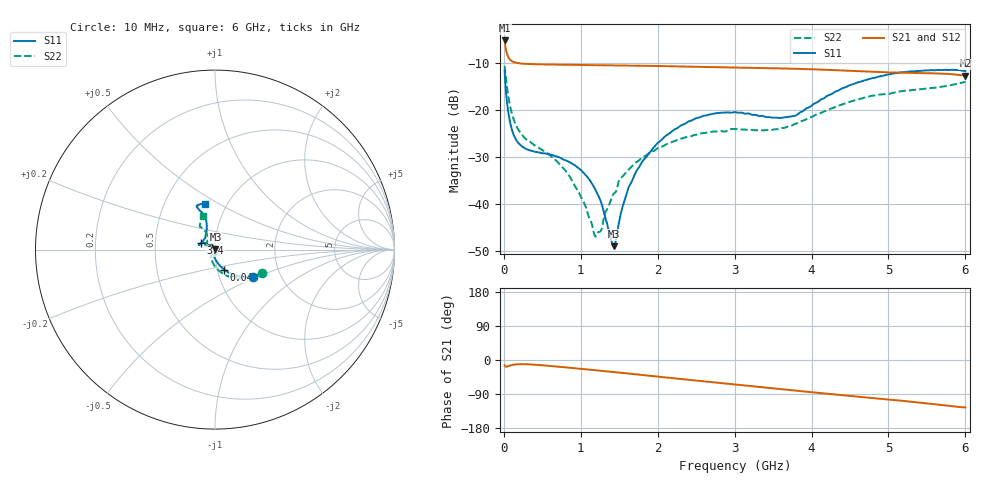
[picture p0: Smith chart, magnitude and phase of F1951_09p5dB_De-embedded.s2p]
! Integrated Device Technology
! Corporate Headquarters
! 6024 Silver Creek Valley Road
! San Jose, CA 95138  USA
! Phone:  1-408-284-8200
! Toll Free:  1-800-223-1366
! Webpage:  http://www.idt.com/
! Timing and RF Division
! 515 Groton Road, Suite 102
! Westford, MA 01886-6024
! Device:  F1951
! Description: 6-bit 0.5 dB Digital Step Attenuator
! Frequency:  100.0 -  4000.00 MHz
! Package:  4x4 mm Thin QFN Plastic Package: 24 pin
! Ports:  2 RF, 6 DC
!  Pin  1  = NC
!  Pin  2  = RF1  =  Port 1
!  Pin  3  = GND
!  Pin  4  = NC
!  Pin  5  = Serial Data Out (SDO)
!  Pin  6  = NC
!  Pin  7  = Reset Bar ( RSTb)
!  Pin  8  = Clock (CLK)
!  Pin  9  = Chip Select Bar (CSb)
!  Pin 10  = NC
!  Pin 11  = Serial Data In (SDI)
!  Pin 12  = NC
!  Pin 13  = NC
!  Pin 14  = VDD
!  Pin 15  = NC
!  Pin 16  = GND
!  Pin 17  = RF2  =  Port 2
!  Pin 18  = NC
!  Pin 19  = GND
!  Pin 20  = GND
!  Pin 21  = GND
!  Pin 22  = GND
!  Pin 23  = GND
!  Pin 24  = GND
! State:  19
! Atten State:  9.5 dB
! Voltage:  +3.30 Volts
! Current:  0.487 mA
! Data:  The device was measured on a F195X evaluation board which has
!  individual transmission lines to the RF pins.  Data was collected
!  de-embedded using a Automatic Fixture Removal [AFR] (Keysight Technologies).
!  The reference plane is the edge of the package pin.
! Misc:  Lot Code  1225BCA
!  Action Tracker AT0399
! Date Measured:  2018-09-13
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# GHz S dB R 50
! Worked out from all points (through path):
!   600 points, 10 MHz to 6 GHz, reference 50 ohm
!   highest |S21| = -5.26 dB at 10 MHz (marker M1); lowest = -12.7 dB at 6 GHz (marker M2)
!   group delay of S21, straight-line fit = 55.5 ps
!   lowest |S11| = -49.0 dB at 1.43 GHz (marker M3), VSWR 1.01, Z = 50.3 + j0.242 ohm
!   |S11| at or under -10 dB: start of sweep to end of sweep
!   |S22| runs from -46.9 to -10.6 dB; largest |S21 - S12| = 0.00048
!   S11 on the Smith chart (normalised r, x): 10 MHz: 1.45, -0.48; 40 MHz: 1.08, -0.24; 3.4 GHz: 0.86, +0.06; 6 GHz: 0.79, +0.43
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0.01  -11.59 -36.0  -5.26 -13.8  -5.26 -13.8  -10.63 -26.6
0.04  -18.23 -65.3  -8.02 -17.5  -8.02 -17.6  -15.05 -60.5
0.07  -21.68 -76.5  -9.12 -15.4  -9.12 -15.4  -18.27 -78.5
0.11  -24.49 -84.7  -9.71 -12.9  -9.71 -12.9  -21.11 -92.5
0.21  -27.39 -94.5  -10.13 -11.0  -10.13 -11.0  -24.72 -110.4
0.76  -30.43 -82.7  -10.41 -18.5  -10.41 -18.6  -32.15 -121.7
1.01  -32.91 -68.7  -10.47 -23.4  -10.48 -23.4  -38.77 -121.6
1.2  -37.29 -56.0  -10.50 -27.1  -10.50 -27.1  -46.75 -177.2
1.26  -39.46 -48.5  -10.51 -28.3  -10.51 -28.3  -45.74 151.6
1.39  -47.37 -1.1  -10.53 -31.0  -10.53 -31.0  -39.22 119.7
1.43  -48.96 42.5  -10.55 -31.9  -10.55 -31.9  -37.76 118.2
1.63  -36.22 113.8  -10.58 -35.9  -10.58 -36.0  -32.58 116.0
1.8  -30.98 125.4  -10.62 -39.6  -10.62 -39.6  -30.10 120.1
2.01  -26.89 136.8  -10.69 -44.0  -10.69 -44.0  -28.06 127.7
2.49  -21.83 153.0  -10.84 -54.1  -10.84 -54.1  -25.31 144.4
3.01  -20.51 162.8  -11.03 -64.7  -11.03 -64.7  -24.05 152.0
3.4  -21.51 155.3  -11.13 -72.7  -11.13 -72.7  -24.31 141.3
3.77  -21.31 128.3  -11.28 -80.4  -11.28 -80.4  -23.10 125.2
4.01  -18.97 114.7  -11.38 -85.3  -11.38 -85.3  -21.46 119.0
4.5  -14.75 106.9  -11.71 -95.1  -11.71 -95.1  -18.29 119.1
5.01  -12.48 111.8  -12.05 -104.5  -12.05 -104.4  -16.59 123.0
6  -11.74 102.9  -12.73 -125.2  -12.73 -125.2  -14.04 109.7
